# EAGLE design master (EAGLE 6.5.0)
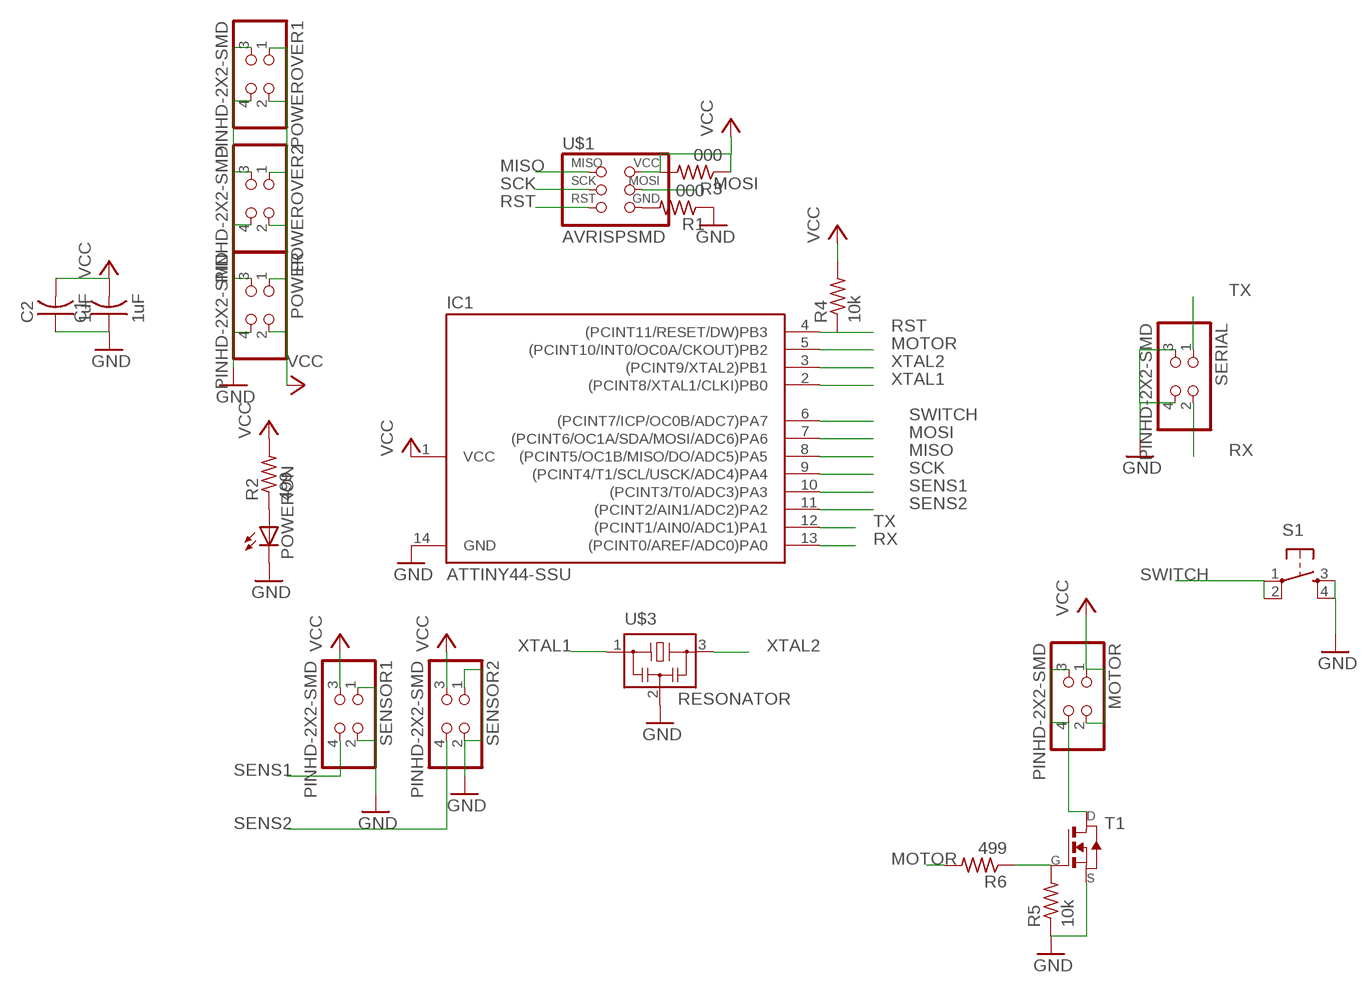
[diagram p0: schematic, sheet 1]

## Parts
C1  1uF  CAP-US1206FAB  [C1206FAB]
C2  1uF  CAP-US1206FAB  [C1206FAB]
IC1  ATTINY44-SSU  [SOIC14]
MOTOR  PINHD-2X2-SMD  [2X02SMD]
POWER  PINHD-2X2-SMD  [2X02SMD]
POWERON  LED1206  [1206]
POWEROVER1  PINHD-2X2-SMD  [2X02SMD]
POWEROVER2  PINHD-2X2-SMD  [2X02SMD]
R1  000  RES-US1206FAB  [R1206FAB]
R2  499  RES-US1206FAB  [R1206FAB]
R3  000  RES-US1206FAB  [R1206FAB]
R4  10k  RES-US1206FAB  [R1206FAB]
R5  10k  RES-US1206FAB  [R1206FAB]
R6  499  RES-US1206FAB  [R1206FAB]
S1  6MM_SWITCH6MM_SWITCH  [6MM_SWITCH]
SENSOR1  PINHD-2X2-SMD  [2X02SMD]
SENSOR2  PINHD-2X2-SMD  [2X02SMD]
SERIAL  PINHD-2X2-SMD  [2X02SMD]
T1  NMOSFETSOT23  [SOT-23]
U$1  AVRISPSMD  [2X03SMD]
U$3  RESONATOR  [EFOBM]

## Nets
GATE: R5.2 R6.1 T1.3(G)
GND: C1.1 C2.1 IC1.14(GND) POWER.3 POWER.4 POWERON.2(C) POWEROVER1.3 POWEROVER1.4 POWEROVER2.3 POWEROVER2.4 R1.1 R5.1 S1.3(S) S1.4(S1) SENSOR1.1 SENSOR1.2 SENSOR2.1 SENSOR2.2 SERIAL.3 SERIAL.4 T1.2(S) U$3.2
MISO: IC1.8((PCINT5/OC1B/MISO/DO/ADC5)PA5) U$1.1(MISO)
MOSI: IC1.7((PCINT6/OC1A/SDA/MOSI/ADC6)PA6) U$1.4(MOSI)
MOTOR: IC1.5((PCINT10/INT0/OC0A/CKOUT)PB2) R6.2
N$1: POWERON.1(A) R2.1
N$2: MOTOR.3 MOTOR.4 T1.1(D)
N$3: R1.2 U$1.6(GND)
RST: IC1.4((PCINT11/RESET/DW)PB3) R4.1 U$1.5(RST)
RX: IC1.13((PCINT0/AREF/ADC0)PA0) SERIAL.2
SCK: IC1.9((PCINT4/T1/SCL/USCK/ADC4)PA4) U$1.3(SCK)
SENS1: IC1.10((PCINT3/T0/ADC3)PA3) SENSOR1.4
SENS2: IC1.11((PCINT2/AIN1/ADC2)PA2) SENSOR2.4
SWITCH: IC1.6((PCINT7/ICP/OC0B/ADC7)PA7) S1.1(P) S1.2(P1)
TX: IC1.12((PCINT1/AIN0/ADC1)PA1) SERIAL.1
VCC: C1.2 C2.2 IC1.1(VCC) MOTOR.1 MOTOR.2 POWER.1 POWER.2 POWEROVER1.1 POWEROVER1.2 POWEROVER2.1 POWEROVER2.2 R2.2 R3.1 R3.2 R4.2 SENSOR1.3 SENSOR2.3 U$1.2(VCC)
XTAL1: IC1.2((PCINT8/XTAL1/CLKI)PB0) U$3.1
XTAL2: IC1.3((PCINT9/XTAL2)PB1) U$3.3

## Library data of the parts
C1 C2 = fab:CAP-US
IC1 = fab:ATTINY44
MOTOR POWER POWEROVER1 POWEROVER2 SENSOR1 SENSOR2 SERIAL = fab:PINHD-2X2-SMD
POWERON = FabLab:LED
R1-R6 = fab:RES-US: Resistor (US Symbol)
S1 = fab:6MM_SWITCH: OMRON SWITCH
T1 = fab:NMOSFET: MOS FET
U$1 = fab:AVRISP
U$3 = fab:RESONATOR

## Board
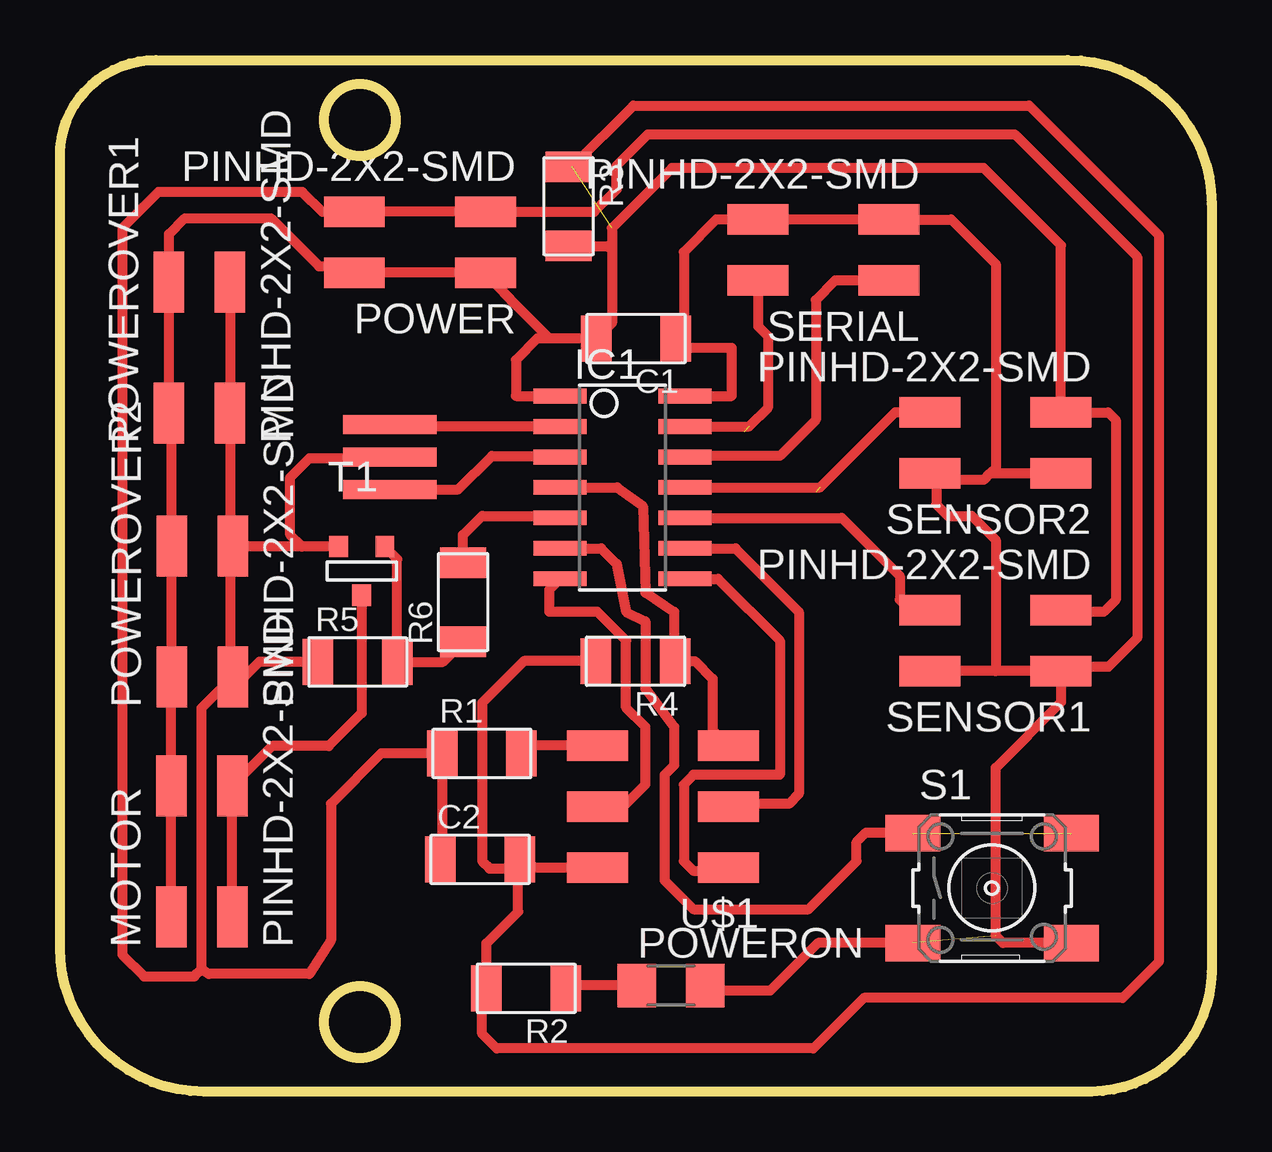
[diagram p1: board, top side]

Size 48 x 43 mm. Coordinates in mm from the lower left corner, seen from the top.
Outline: 42,43 arc-90 48,37 48,5 arc-90 43,0 6,0 arc-90 0,6 0,39 arc-90 4,43 42,43
Outline: circle at 12.5,2.9 radius 1.5
Outline: circle at 12.5,40.5 radius 1.5
Copper layers (1*16): Top 0.035mm / dielectric 1.5mm / Bottom 0.035mm
Design rules "default": minimum track width 10mil, minimum drill 24mil, track to track 8mil, track to pad 8mil, pad to pad 8mil, via to via 8mil, smd to smd 8mil, copper to edge 40mil, drill to drill 8mil, minimum pad ring 10mil, minimum via ring 8mil, stop-mask expansion 4mil, vias tented up to drill 0mil, thermal gap 10mil

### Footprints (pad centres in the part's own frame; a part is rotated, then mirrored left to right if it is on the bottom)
C1206FAB = smd 1.27 x 1.905: 1 -1.651,0; 2 1.651,0
SOIC14 = smd 0.61 x 2.21: 1 -3.81,-2.603; 2 -2.54,-2.603; 3 -1.27,-2.603; 4 0,-2.603; 5 1.27,-2.603; 6 2.54,-2.603; 7 3.81,-2.603; 8 3.81,2.603; 9 2.54,2.603; 10 1.27,2.603; 11 0,2.603; 12 -1.27,2.603; 13 -2.54,2.603; 14 -3.81,2.603
2X02SMD = smd 2.54 x 1.27: 1 -2.54,1.27; 2 2.92,1.27; 3 -2.54,-1.27; 4 2.92,-1.27
1206 = smd 1.6 x 1.803: 1 -1.422,0; 2 1.422,0
R1206FAB = smd 1.27 x 1.905: 1 -1.651,0; 2 1.651,0
6MM_SWITCH = smd 2.286 x 1.524: 1 -3.302,2.286; 2 3.302,2.286; 3 -3.302,-2.286; 4 3.302,-2.286
SOT-23 = smd 0.787 x 0.889: 1 0.025,-1.016; 2 -0.94,1.016; 3 0.991,1.016
2X03SMD = smd 2.54 x 1.27: 1 -2.54,2.54; 2 2.92,2.54; 3 -2.54,0; 4 2.92,0; 5 -2.54,-2.54; 6 2.92,-2.54
EFOBM = smd 0.8 x 3.9: 1 -1.35,0; 2 0,0; 3 1.35,0

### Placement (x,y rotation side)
C1  24.01,31.39 180 top
C2  17.51,9.68 0 top
IC1  23.45,25.18 270 top
MOTOR  5.91,9.82 90 top
POWER  15.19,35.4 180 top
POWERON  25.47,4.42 0 top
POWEROVER1  5.82,30.82 90 top
POWEROVER2  5.93,19.82 90 top
R1  17.58,14.09 0 top
R2  19.43,4.3 180 top
R3  21.2,36.9 270 top
R4  23.99,17.94 180 top
R5  12.41,17.91 0 top
R6  16.8,20.4 90 top
S1  38.85,8.48 0 top
SENSOR1  39.18,18.8 180 top
SENSOR2  39.18,27.04 180 top
SERIAL  32.02,35.08 180 top
T1  12.55,21.7 0 top
U$1  25.32,11.88 180 top
U$3  13.75,26.45 270 top

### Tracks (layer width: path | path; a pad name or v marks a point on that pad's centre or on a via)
GATE
  Top 0.406: R6.1 15.96,17.91 R5.2 14.06,22.2 T1.3
GND  (1 unrouted)
  Top 0.406: IC1.14 27.99,28.99 28,29 28,31 26.05,31 C1.1 26,31.73 26,35 27.35,36.35 SERIAL.4 SERIAL.3 37.15,36.35 39,34.5 39,26 38.77,25.77 | 38.77,25.77 38.5,25.5 36.53,25.5 | 36.53,25.5 SENSOR2.2 | SENSOR2.1 38.77,25.77 | SENSOR1.1 39,17.53 | 39,17.53 SENSOR1.2 | 36.53,25.5 36.53,24.47 37,24 38,24 39,23 39,17.53 | SENSOR1.1 41.72,16.22 39,13.5 39,6.5 39.31,6.19 S1.4 42,6.04 | 15.8,10.04 C2.1 15.93,9.75 R1.1 13.39,14.09 11.3,12 11.3,6.3 10.4,4.9 6.2,4.9 5.9,5.1 | S1.3 31.59,6.19 29.6,4.2 26.67,4.2 | 26.3,4.2 26.67,4.2 | 26.67,4.2 POWERON.2 | 5.9,5.1 5.6,4.8 3.5,4.8 2.6,5.7 2.6,36 4.1,37.5 10.1,37.5 10.93,36.67 POWER.4 POWER.3 22.27,36.67 23.2,37.6 23.2,38.6 24.5,39.9 39.8,39.9 44.9,34.8 44.9,18.9 43.7,17.7 41.89,17.7 SENSOR1.1 | 5.9,5.1 5.9,15.98 POWEROVER2.3 | R5.1 8.31,17.91 7.2,16.8 POWEROVER2.3 | U$3.2 13.7,26.4 10.4,26.4 9.6,25.6 9.6,23.2 10.08,22.72 T1.2 11.59,22.74 POWEROVER2.4 7.09,22.85 POWEROVER1.3 POWEROVER1.4 7.09,17.39 POWEROVER2.3
MISO
  Top 0.406: IC1.8 27.43,21.37 30,18.8 30,13.2 26.4,13.2 26,12.8 26,9.6 26.4,9.2 27.72,9.2 U$1.1
MOSI
  Top 0.406: U$1.4 23.48,11.88 24.4,12.8 24.4,15.2 23.6,16 23.6,18.8 22.4,20 20.4,20 20.4,20.92 IC1.7
MOTOR
  Top 0.406: R6.2 16.8,23.2 17.6,24 20.76,24 IC1.5
N$1
  Top 0.406: POWERON.1 21.2,4.42 R2.1
N$2
  Top 0.406: MOTOR.3 MOTOR.4 8.84,14.4 11.2,14.4 12.58,15.77 T1.1
N$3
  Top 0.406: U$1.6 19.56,14.42 R1.2
RST
  Top 0.406: IC1.4 23.22,25.18 24.3,24.4 24.4,20.8 25.6,20 25.6,17.98 R4.1 26.46,17.94 27.2,17.2 27.2,15.08 U$1.5
RX  (1 unrouted)
  Top 0.406: SERIAL.2 29.1,31.9 29.5,31.5 29.5,28.5 28.72,27.72 IC1.13
SCK
  Top 0.406: IC1.9 28.16,22.64 30.8,20 30.8,12.4 30.4,12 27.98,12 U$1.3
SENS1
  Top 0.406: IC1.10 32.59,23.91 35,21.5 35,20.5 35.5,20 36.19,20 SENSOR1.4
SENS2  (1 unrouted)
  Top 0.406: SENSOR2.4 34.81,28.31 31.68,25.18 IC1.11
SWITCH  (1 unrouted)
  Top 0.406: IC1.6 22.56,22.64 23.2,22 23.6,20 24.4,19.6 24.4,16.8 25.6,15.2 25.6,13.6 25.2,13.2 25.2,8.8 26.4,7.6 31.2,7.6 33.2,9.6 33.2,10.4 33.6,10.8 35.51,10.8 S1.1
TX
  Top 0.406: SERIAL.1 32.31,33.81 31.5,33 31.5,28 30,26.5 26.1,26.5 IC1.12
VCC  (1 unrouted)
  Top 0.406: SENSOR1.3 41.79,20 43.5,20 44,20.5 44,28 43.69,28.31 SENSOR2.3 41.72,35.28 38.5,38.5 25.5,38.5 23,36 23,35.1 | 23,35.1 23,32.03 C1.2 20.4,31.39 | 20.4,31.39 19.89,31.39 19,30.5 19,29 20.84,29 IC1.1 | MOTOR.1 MOTOR.2 4.64,17.26 POWEROVER2.1 POWEROVER2.2 4.66,28.17 POWEROVER1.1 POWEROVER1.2 4.55,35.75 5.2,36.4 8.8,36.4 10.8,34.4 13.2,34.4 POWER.2 POWER.1 18.93,32.86 20.4,31.39 | C2.2 19.8,9.34 U$1.2 | C2.2 19.1,9.92 19.1,7.5 17.78,6.18 R2.2 17.6,4.12 17.6,2.4 18.2,1.8 31.4,1.8 33.5,3.9 44.3,3.9 45.8,5.4 45.8,35.7 40.4,41.1 23.9,41.1 21.35,38.55 R3.1 | R3.2 22.85,35.25 23,35.1 | R4.2 19.34,17.94 17.6,16.2 17.6,9.6 17.9,9.3 18.78,9.3 C2.2
XTAL1
  Top 0.406: IC1.2 13.83,27.72 U$3.1
XTAL2
  Top 0.406: U$3.3 16.6,25.1 18,26.5 20.8,26.5 IC1.3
